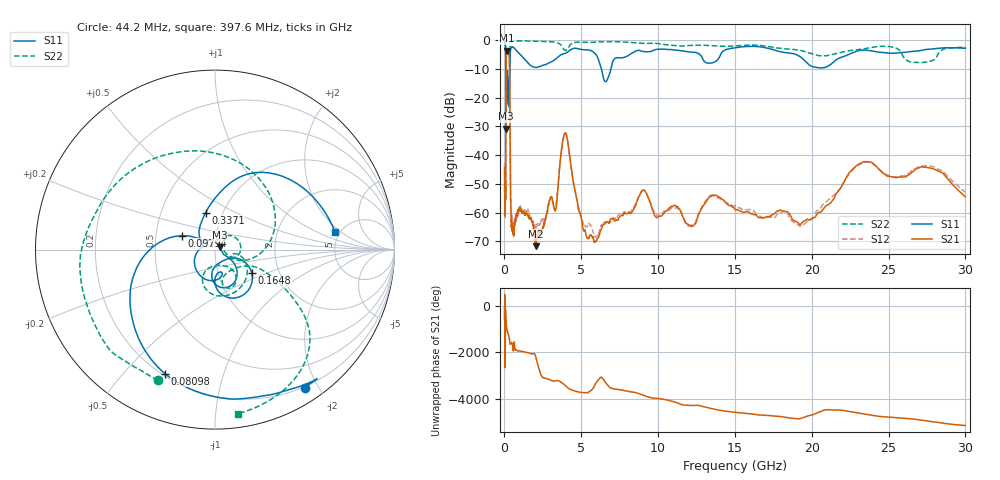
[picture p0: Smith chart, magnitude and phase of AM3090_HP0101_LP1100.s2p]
! Date/Time: Thu, Feb 28, 2019 1:59 PM
! Network Analyzer: Agilent Technologies E8364B Rev: A.07.50.67
! Sweep from 0.010 to 30.000 GHz, 1601 Points, Sweep Type: LOG
! Power Supply: 5.023 V, 0.002 A
# Hz S DB R 50
!freq MagS11 AngS11 MagS21 AngS21 MagS12 AngS12 MagS22 AngS22
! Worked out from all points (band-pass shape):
!   1601 points, 10 MHz to 30 GHz, reference 50 ohm
!   highest |S21| = -3.71 dB at 161.5 MHz (marker M1); lowest = -71.7 dB at 2.042 GHz (marker M2)
!   |S21| within 3 dB of the highest: 108.6 MHz to 320.6 MHz (212 MHz wide, 98.8 % of centre)
!   lowest |S11| = -30.8 dB at 105.6 MHz (marker M3), VSWR 1.06, Z = 52.6 + j1.36 ohm
!   |S11| at or under -10 dB: 95.93 MHz to 349.6 MHz (253.6 MHz wide, 114 % of centre); 6.308 GHz to 6.931 GHz (622.7 MHz wide, 9.41 % of centre)
!   |S22| runs from -28.3 to -0.1 dB; largest |S21 - S12| = 0.012
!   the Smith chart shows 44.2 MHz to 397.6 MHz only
!   S11 on the Smith chart (normalised r, x): 44.2 MHz: 0.19, -1.83; 80.98 MHz: 0.21, -0.65; 97.94 MHz: 0.68, +0.11; 164.8 MHz: 1.45, -0.40; 337.1 MHz: 0.83, +0.36; 397.6 MHz: 4.56, +1.63
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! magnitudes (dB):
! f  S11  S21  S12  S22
! 10 MHz  -0.2  -44.4  -47.4  -0.7
! 38.04 MHz  -0.5  -58.5  -59.7  -1.5
! 44.2 MHz  -0.7  -55.3  -56.0  -2.0
! 80.98 MHz  -2.6  -49.1  -47.4  -4.7
! 97.94 MHz  -13.9  -14.5  -14.5  -13.5
! 105.6 MHz  -30.8  -7.7  -7.7  -27.9
! 120.2 MHz  -13.3  -5.1  -5.1  -17.8
! 144.7 MHz  -22.3  -3.9  -3.9  -20.3
! 161.5 MHz  -13.2  -3.7  -3.7  -15.7
! 164.8 MHz  -12.3  -3.7  -3.7  -14.7
! 337.1 MHz  -13.5  -10.0  -10.0  -8.4
! 397.6 MHz  -3.4  -53.9  -53.2  -0.7
! 550.5 MHz  -2.5  -66.3  -63.9  -0.2
! 2.042 GHz  -9.5  -71.7  -65.1  -0.4
! 2.084 GHz  -9.5  -70.6  -64.3  -0.4
! 3.318 GHz  -6.7  -59.1  -58.9  -0.8
! 3.934 GHz  -4.6  -32.3  -32.4  -3.6
! 5.285 GHz  -3.4  -67.1  -65.0  -0.8
! 7.926 GHz  -5.7  -60.4  -59.9  -0.7
! 19.31 GHz  -6.0  -63.9  -64.6  -3.6
! 23.48 GHz  -3.5  -42.2  -42.4  -3.0
! 30 GHz  -2.8  -54.5  -52.9  -2.5
